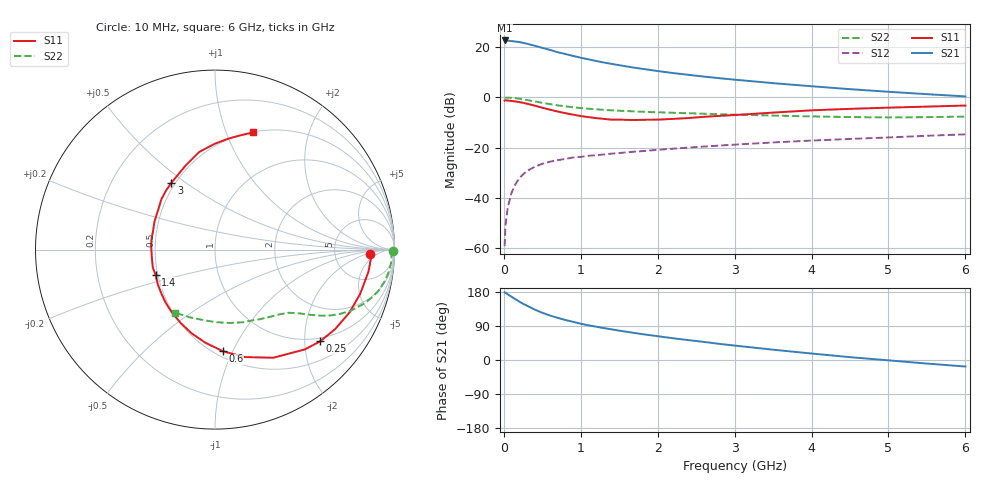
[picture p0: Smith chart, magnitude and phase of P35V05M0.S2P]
! SIEMENS Small Signal Semiconductors
! BFP181
! Si NPN RF Bipolar Junction Transistor in SOT143
! VCE = 5 V  IC = 5 mA
! Common Emitter S-Parameters:  March  1996
# GHz  S  MA  R  50
!  f  S11  S21  S12  S22
! GHz  MAG  ANG  MAG  ANG  MAG  ANG  MAG  ANG
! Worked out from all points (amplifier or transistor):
!   36 points, 10 MHz to 6 GHz, reference 50 ohm
!   highest |S21| = 22.6 dB at 10 MHz (marker M1)
!   |S21| within 3 dB of that: start of sweep to 505.5 MHz
!   unconditionally stable (mu >= 1): 1.759 GHz to end of sweep
!   at 250 MHz: K = 0.21, MSG = 26.1 dB, |S12| = -30.6 dB
!   at 1.4 GHz: K = 0.89, MSG = 17.8 dB, |S12| = -22.4 dB
!   at 6 GHz: K = 1.05, MAG = 6.2 dB, |S12| = -14.7 dB
!   lowest NFmin = 1.55 dB at 450 MHz
!   S11 on the Smith chart (normalised r, x): 10 MHz: 13, -3; 250 MHz: 0.91, -2.36; 600 MHz: 0.55, -0.92; 1.4 GHz: 0.49, -0.16; 3 GHz: 0.48, +0.44; 6 GHz: 0.51, +1.25
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0.01  0.8614 -1.8  13.48 178.3  0.0011 86.7  0.9911 -0.6
0.02  0.8701 -3.3  13.4 177.5  0.0027 77.3  0.9838 -1.4
0.05  0.8638 -8.2  13.34 173.3  0.0064 88.1  0.986 -3.7
0.1  0.8455 -17.0  13.09 166.9  0.0127 78.7  0.9759 -7.4
0.2  0.8027 -33.5  12.55 154.3  0.0245 73.0  0.939 -14.2
0.25  0.7774 -41.1  12.07 148.3  0.0294 68.6  0.9116 -17.2
0.3  0.7478 -48.1  11.61 143.5  0.0343 64.7  0.885 -19.8
0.4  0.6843 -61.7  10.61 133.2  0.0415 59.0  0.8301 -24.2
0.5  0.6213 -74.5  9.593 124.6  0.0477 54.2  0.7779 -27.6
0.6  0.5683 -85.5  8.755 117.4  0.0526 50.4  0.7315 -30.2
0.7  0.5213 -96.0  7.868 111.2  0.0562 47.9  0.6921 -32.1
0.8  0.4842 -105.6  7.24 105.6  0.0598 46.0  0.6614 -33.5
1  0.4245 -124.5  6.107 95.8  0.0654 43.3  0.6119 -35.9
1.1  0.4032 -133.2  5.69 91.5  0.0688 41.9  0.5924 -36.9
1.4  0.3595 -156.8  4.617 80.9  0.0759 40.2  0.5514 -39.8
1.8  0.3567 176.1  3.679 68.2  0.0852 38.8  0.5165 -43.9
2.2  0.3722 154.8  3.032 57.4  0.0952 37.0  0.4926 -48.7
3  0.4444 123.2  2.241 38.1  0.1146 33.3  0.4512 -60.1
3.5  0.4967 109.2  1.911 27.2  0.1267 30.9  0.4342 -68.8
4.5  0.5894 90.2  1.451 7.5  0.1488 24.5  0.4047 -89.1
5.5  0.653 77.3  1.154 -9.4  0.1719 18.9  0.4034 -110.9
6  0.6861 72.0  1.042 -17.2  0.1837 15.3  0.4143 -122.1
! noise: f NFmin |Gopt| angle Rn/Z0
0.45  1.55  0.48  17  0.36
0.9  1.65  0.4  35  0.34
1.8  2  0.18  88  0.34
